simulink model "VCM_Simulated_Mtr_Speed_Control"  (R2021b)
settings: Solver=VariableStepAuto  StartTime=0.0  StopTime=5  MaxStep=1e-4  RelTol=1e-3
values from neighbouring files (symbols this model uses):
  FluidProp = struct    [HydMtrCtrlSys_paramsV1.m]    (also in HydMtrCtrlSys_paramsV2.m)
  Motor = struct    [HydMtrCtrlSys_paramsV1.m]    (also in HydMtrCtrlSys_paramsV2.m)
  MotorInletVolume = struct    [HydMtrCtrlSys_paramsV1.m]    (also in HydMtrCtrlSys_paramsV2.m)
  Pump = struct    [HydMtrCtrlSys_paramsV1.m]    (also in HydMtrCtrlSys_paramsV2.m)
  ReturnPressure_psi = 30    [HydMtrCtrlSys_paramsV1.m]    (also in HydMtrCtrlSys_paramsV2.m)
  SupplyVolume = struct    [HydMtrCtrlSys_paramsV1.m]    (also in HydMtrCtrlSys_paramsV2.m)
  SystemVolume = struct    [HydMtrCtrlSys_paramsV1.m]    (also in HydMtrCtrlSys_paramsV2.m)
  Valve1 = struct    [HydMtrCtrlSys_paramsV1.m]    (also in HydMtrCtrlSys_paramsV2.m)
libraries: simulink x5

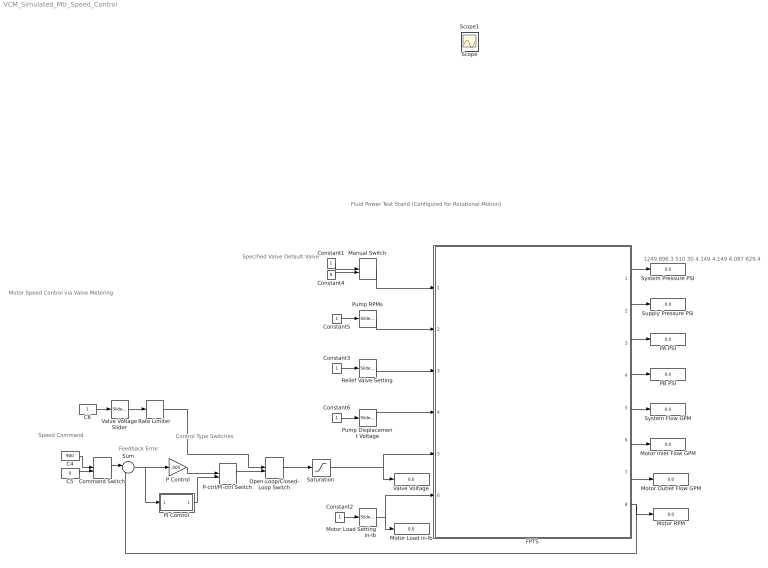
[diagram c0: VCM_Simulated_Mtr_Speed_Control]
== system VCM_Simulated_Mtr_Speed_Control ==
  note: 1249 896.3 510 30 4.149 4.149 4.087 629.4
  note: Fluid Power Test Stand (Configured for Rotational Motion)
  note: Specified Valve Default Valve
  note: Control Type Switches
  note: Speed Command
  note: Feedback Error
  note: Motor Speed Control via Valve Metering
  C4 : Constant  Value=900
  C5 : Constant  Value=0
  C6 : Constant
  Command Switch : ManualSwitch
  Constant{1..3,5..6} (5 alike) : Constant
  Constant4 : Constant  Value=0
  FPTS : Subsystem
  Manual Switch : ManualSwitch  CurrentSetting=0
  Motor Load Setting in-lb : simulink/Math Operations/Slider Gain  gain=80.0  low=80  high=250
  Motor Inlet Flow GPM : Display
  Motor Load in-lb : Display
  Motor Outlet Flow GPM : Display
  Motor RPM : Display
  Open-Loop/Closed-Loop Switch : ManualSwitch
  P Control : Gain  Gain=.005
  P-ctrl/PI-ctrl Switch : ManualSwitch
  PA PSI : Display
  PB PSI : Display
  PI Control : Subsystem
  Pump Displacement Voltage : simulink/Math Operations/Slider Gain  gain=0.0  low=0  high=5
  Pump RPMs : simulink/Math Operations/Slider Gain  gain=0.0  low=0  high=1200
  Rate Limiter : RateLimiter  SampleTimeMode=inherited
  Relief Valve Setting : simulink/Math Operations/Slider Gain  gain=0.0  low=0  high=5
  Saturation : Saturate  UpperLimit=10  LowerLimit=-10
  Sum : Sum  Inputs=|+-
  Supply Pressure PSI : Display
  System Flow GPM : Display
  System Pressure PSI : Display
  Valve Voltage : Display
  Valve Voltage Slider : simulink/Math Operations/Slider Gain  gain=0.0  low=0  high=10
  Scope : Scope
  Scope1 : Scope
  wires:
  Constant3/1 -> Relief Valve Setting/1
  PI Control/1(Ctrl) -> P-ctrl/PI-ctrl Switch/2
  Rate Limiter/1 -> Open-Loop/Closed-Loop Switch/1
  P-ctrl/PI-ctrl Switch/1 -> Open-Loop/Closed-Loop Switch/2
  C6/1 -> Valve Voltage Slider/1
  C5/1 -> Command Switch/2
  P Control/1 -> P-ctrl/PI-ctrl Switch/1
  Sum/1 -> P Control/1, PI Control/1(Err)
  C4/1 -> Command Switch/1
  Valve Voltage Slider/1 -> Rate Limiter/1
  Open-Loop/Closed-Loop Switch/1 -> Saturation/1
  Command Switch/1 -> Sum/1
  Constant1/1 -> Manual Switch/1
  Constant2/1 -> Motor Load Setting in-lb/1
  Motor Load Setting in-lb/1 -> Motor Load in-lb/1, FPTS/6(Load Torque)
  Saturation/1 -> Valve Voltage/1, FPTS/5(valve_signal_V)
  Constant4/1 -> Manual Switch/2
  Constant6/1 -> Pump Displacement Voltage/1
  Constant5/1 -> Pump RPMs/1
  FPTS/8(rpm) -> Sum/2, Motor RPM/1
  Relief Valve Setting/1 -> FPTS/3(set_PRV)
  Manual Switch/1 -> FPTS/1(set_valve)
  Pump Displacement Voltage/1 -> FPTS/4(pump_signal_V)
  Pump RPMs/1 -> FPTS/2(pump_rpm)
  FPTS/1(Psys_psi) -> System Pressure PSI/1
  FPTS/2(PV_psi) -> Supply Pressure PSI/1
  FPTS/3(PA_psi) -> PA PSI/1
  FPTS/4(PB_psi) -> PB PSI/1
  FPTS/5(QS_gpm) -> System Flow GPM/1
  FPTS/6(QMI_gpm) -> Motor Inlet Flow GPM/1
  FPTS/7(QMO_gpm) -> Motor Outlet Flow GPM/1

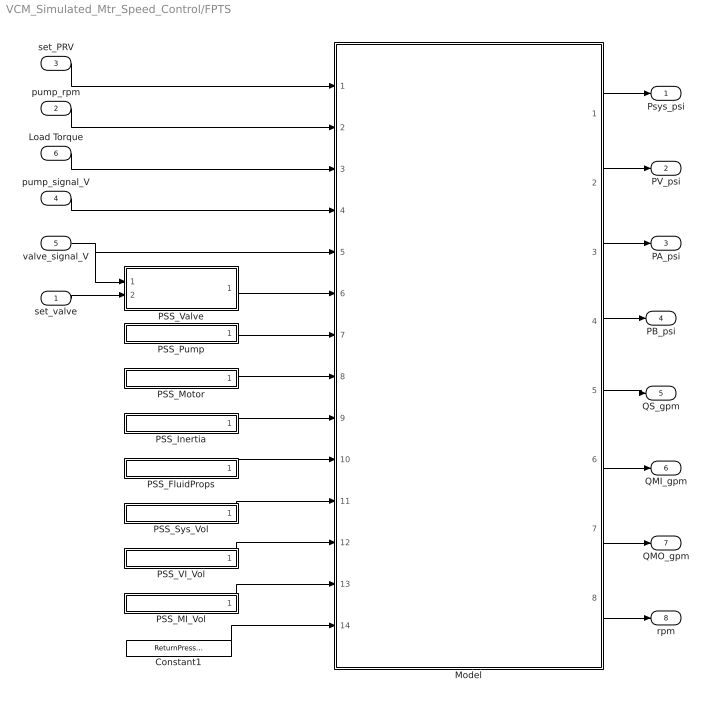
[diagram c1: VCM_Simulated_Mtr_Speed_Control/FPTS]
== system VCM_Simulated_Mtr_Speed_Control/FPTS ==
  set_valve : Inport
  pump_rpm : Inport  Port=2
  set_PRV : Inport  Port=3
  pump_signal_V : Inport  Port=4
  valve_signal_V : Inport  Port=5
  Load Torque : Inport  Port=6
  Constant1 : Constant  Value=ReturnPressure_psi
  Model : ModelReference  ModelNameDialog=FPTS_VCMM_v3_21b.slxp  ModelReferenceVersion=4.38  CopyOfModelProtected=on
  PSS_FluidProps : Subsystem
  PSS_Inertia : Subsystem
  PSS_MI_Vol : Subsystem
  PSS_Motor : Subsystem
  PSS_Pump : Subsystem
  PSS_Sys_Vol : Subsystem
  PSS_VI_Vol : Subsystem
  PSS_Valve : Subsystem
  Psys_psi : Outport
  PV_psi : Outport  Port=2
  PA_psi : Outport  Port=3
  PB_psi : Outport  Port=4
  QS_gpm : Outport  Port=5
  QMI_gpm : Outport  Port=6
  QMO_gpm : Outport  Port=7
  rpm : Outport  Port=8
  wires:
  Model/1 -> Psys_psi/1
  Model/7 -> QMO_gpm/1
  set_PRV/1 -> Model/1
  Model/8 -> rpm/1
  Model/4 -> PB_psi/1
  Model/3 -> PA_psi/1
  Model/6 -> QMI_gpm/1
  Model/5 -> QS_gpm/1
  Model/2 -> PV_psi/1
  valve_signal_V/1 -> PSS_Valve/1(valve_signal_V), Model/5
  Load Torque/1 -> Model/3
  pump_signal_V/1 -> Model/4
  set_valve/1 -> PSS_Valve/2(set_valve)
  pump_rpm/1 -> Model/2
  PSS_Valve/1(Kv) -> Model/6
  PSS_Pump/1(Pump) -> Model/7
  PSS_Motor/1(Motor) -> Model/8
  PSS_Inertia/1(Inertia) -> Model/9
  PSS_FluidProps/1(Fluid Propserties) -> Model/10
  PSS_MI_Vol/1(Vol) -> Model/13
  PSS_VI_Vol/1(Vol) -> Model/12
  PSS_Sys_Vol/1(Vol) -> Model/11
  Constant1/1 -> Model/14

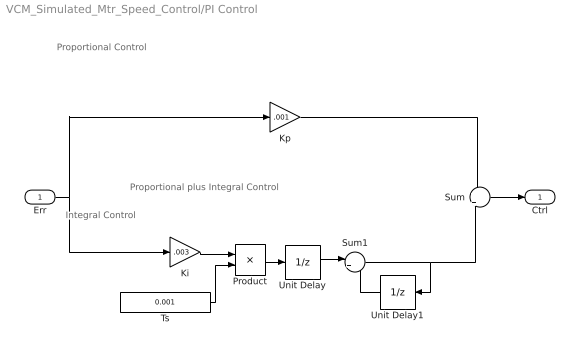
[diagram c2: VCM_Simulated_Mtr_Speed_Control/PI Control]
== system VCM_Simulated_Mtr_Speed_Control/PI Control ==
  note: Proportional plus Integral Control
  note: Proportional Control
  note: Integral Control
  Err : Inport
  Ki : Gain  Gain=.003
  Kp : Gain  Gain=.001
  Product : Product
  Sum : Sum  Inputs=+|+
  Sum1 : Sum  Inputs=|++
  Ts : Constant  Value=0.001
  Unit Delay : UnitDelay  SampleTime=0.001  HasFrameUpgradeWarning=on
  Unit Delay1 : UnitDelay  SampleTime=-1  HasFrameUpgradeWarning=on
  Ctrl : Outport  VectorParamsAs1DForOutWhenUnconnected=off
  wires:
  Sum/1 -> Ctrl/1
  Ki/1 -> Product/1
  Ts/1 -> Product/2
  Err/1 -> Ki/1, Kp/1
  Product/1 -> Unit Delay/1
  Unit Delay/1 -> Sum1/1
  Sum1/1 -> Unit Delay1/1, Sum/2
  Unit Delay1/1 -> Sum1/2
  Kp/1 -> Sum/1

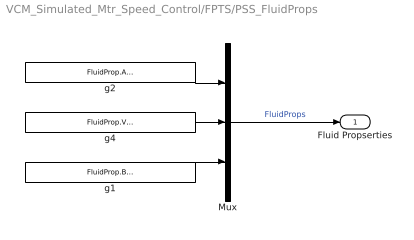
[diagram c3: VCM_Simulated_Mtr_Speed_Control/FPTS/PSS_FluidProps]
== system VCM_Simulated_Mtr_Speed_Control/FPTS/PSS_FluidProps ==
  Mux : Mux  Inputs=3
  g1 : Constant  Value=FluidProp.BulkModulus_psi
  g2 : Constant  Value=FluidProp.Air_0to1
  g4 : Constant  Value=FluidProp.VaporPressure_psi
  Fluid Propserties : Outport
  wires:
  Mux/1 -> Fluid Propserties/1  "FluidProps"
  g4/1 -> Mux/2
  g2/1 -> Mux/1
  g1/1 -> Mux/3

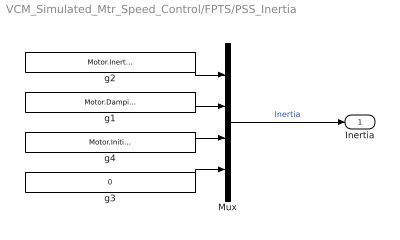
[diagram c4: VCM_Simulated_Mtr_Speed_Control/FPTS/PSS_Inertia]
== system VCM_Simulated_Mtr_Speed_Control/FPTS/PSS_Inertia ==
  Mux : Mux
  g1 : Constant  Value=Motor.Damping_inlbsec
  g2 : Constant  Value=Motor.Inertia_inlbsec2
  g3 : Constant  Value=0
  g4 : Constant  Value=Motor.InitialSpeed_rps
  Inertia : Outport
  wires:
  g2/1 -> Mux/1
  g1/1 -> Mux/2
  g3/1 -> Mux/4
  g4/1 -> Mux/3
  Mux/1 -> Inertia/1  "Inertia"

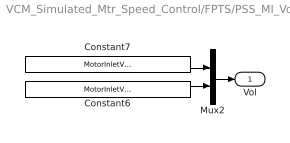
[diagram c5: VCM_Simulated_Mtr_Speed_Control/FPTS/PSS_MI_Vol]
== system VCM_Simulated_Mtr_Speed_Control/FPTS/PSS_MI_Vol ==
  Constant6 : Constant  Value=MotorInletVolume.Init_psi
  Constant7 : Constant  Value=MotorInletVolume.Volume_in3
  Mux2 : Mux  Inputs=2
  Vol : Outport
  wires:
  Constant6/1 -> Mux2/2
  Constant7/1 -> Mux2/1
  Mux2/1 -> Vol/1

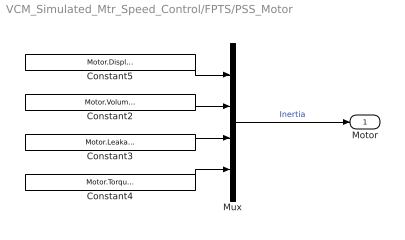
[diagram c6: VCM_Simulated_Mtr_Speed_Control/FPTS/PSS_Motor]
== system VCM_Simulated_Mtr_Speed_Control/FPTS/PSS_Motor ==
  Constant2 : Constant  Value=Motor.VolumetricEff_0to1
  Constant3 : Constant  Value=Motor.LeakageCoeff_in3perpsisec
  Constant4 : Constant  Value=Motor.TorqueEff_0to1
  Constant5 : Constant  Value=Motor.Displacement_in3
  Mux : Mux
  Motor : Outport
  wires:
  Mux/1 -> Motor/1  "Inertia"
  Constant3/1 -> Mux/3
  Constant4/1 -> Mux/4
  Constant2/1 -> Mux/2
  Constant5/1 -> Mux/1

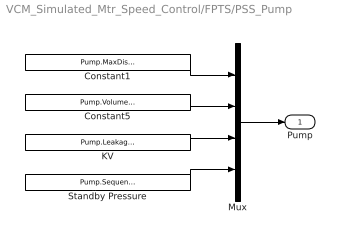
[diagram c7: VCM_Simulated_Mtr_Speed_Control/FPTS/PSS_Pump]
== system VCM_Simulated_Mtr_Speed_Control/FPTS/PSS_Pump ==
  Constant1 : Constant  Value=Pump.MaxDisplacement_in3
  Constant5 : Constant  Value=Pump.VolumetricEff_0to1
  KV : Constant  Value=Pump.LeakageKv
  Mux : Mux
  Standby Pressure : Constant  Value=Pump.SequencePressure_psi
  Pump : Outport
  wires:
  KV/1 -> Mux/3
  Constant1/1 -> Mux/1
  Constant5/1 -> Mux/2
  Mux/1 -> Pump/1
  Standby Pressure/1 -> Mux/4

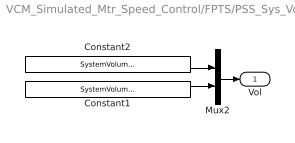
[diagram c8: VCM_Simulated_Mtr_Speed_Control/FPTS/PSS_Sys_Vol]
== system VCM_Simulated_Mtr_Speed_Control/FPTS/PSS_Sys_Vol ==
  Constant1 : Constant  Value=SystemVolume.Init_psi
  Constant2 : Constant  Value=SystemVolume.Volume_in3
  Mux2 : Mux  Inputs=2
  Vol : Outport
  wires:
  Mux2/1 -> Vol/1
  Constant2/1 -> Mux2/1
  Constant1/1 -> Mux2/2

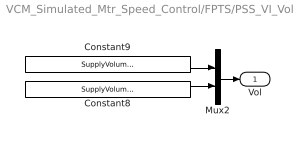
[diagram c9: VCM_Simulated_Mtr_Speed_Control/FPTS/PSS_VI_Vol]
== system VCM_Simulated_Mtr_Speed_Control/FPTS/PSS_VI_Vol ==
  Constant8 : Constant  Value=SupplyVolume.Init_psi
  Constant9 : Constant  Value=SupplyVolume.Volume_in3
  Mux2 : Mux  Inputs=2
  Vol : Outport
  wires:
  Mux2/1 -> Vol/1
  Constant9/1 -> Mux2/1
  Constant8/1 -> Mux2/2

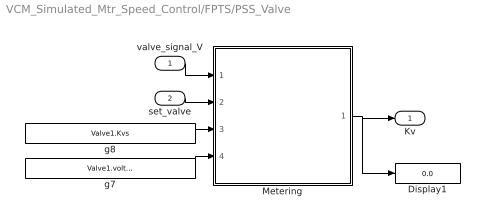
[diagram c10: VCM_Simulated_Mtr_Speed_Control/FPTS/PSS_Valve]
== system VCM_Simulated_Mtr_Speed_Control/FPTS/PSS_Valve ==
  valve_signal_V : Inport
  set_valve : Inport  Port=2
  Display1 : Display
  Metering : Subsystem
  g7 : Constant  Value=Valve1.voltages
  g8 : Constant  Value=Valve1.Kvs
  Kv : Outport
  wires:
  valve_signal_V/1 -> Metering/1(valve_signal_V)
  Metering/1(Out1) -> Kv/1, Display1/1
  g7/1 -> Metering/4(volts)
  g8/1 -> Metering/3(Kvs)
  set_valve/1 -> Metering/2(set_valve)

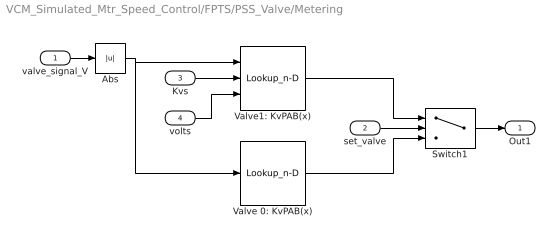
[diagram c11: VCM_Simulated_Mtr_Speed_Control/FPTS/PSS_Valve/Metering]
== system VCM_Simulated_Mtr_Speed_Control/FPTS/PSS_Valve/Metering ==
  valve_signal_V : Inport
  set_valve : Inport  Port=2
  Kvs : Inport  Port=3
  volts : Inport  Port=4
  Abs : Abs
  Switch1 : Switch  Criteria=u2 > Threshold  Threshold=0.5
  Valve 0: KvPAB(x) : Lookup_n-D  NumberOfTableDimensions=1  BreakpointsForDimension1=[-10 0.34 8 9.64 10]  Table=[0 0 1.1 1.2 1.2]  ExtrapMethod=Clip  UseLastTableValue=on  InternalRulePriority=Speed  RndMeth=Simplest
  Valve1: KvPAB(x) : Lookup_n-D  NumberOfTableDimensions=1  BreakpointsForDimension1Source=Input port  BreakpointsForDimension1=Valve1.voltages  TableSource=Input port  Table=Valve1.Kvs  ExtrapMethod=Clip  UseLastTableValue=on  InternalRulePriority=Speed  RndMeth=Simplest
  Out1 : Outport  VectorParamsAs1DForOutWhenUnconnected=off
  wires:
  Valve 0: KvPAB(x)/1 -> Switch1/3
  Valve1: KvPAB(x)/1 -> Switch1/1
  valve_signal_V/1 -> Abs/1
  Switch1/1 -> Out1/1
  set_valve/1 -> Switch1/2
  Abs/1 -> Valve1: KvPAB(x)/1, Valve 0: KvPAB(x)/1
  Kvs/1 -> Valve1: KvPAB(x)/2
  volts/1 -> Valve1: KvPAB(x)/3
